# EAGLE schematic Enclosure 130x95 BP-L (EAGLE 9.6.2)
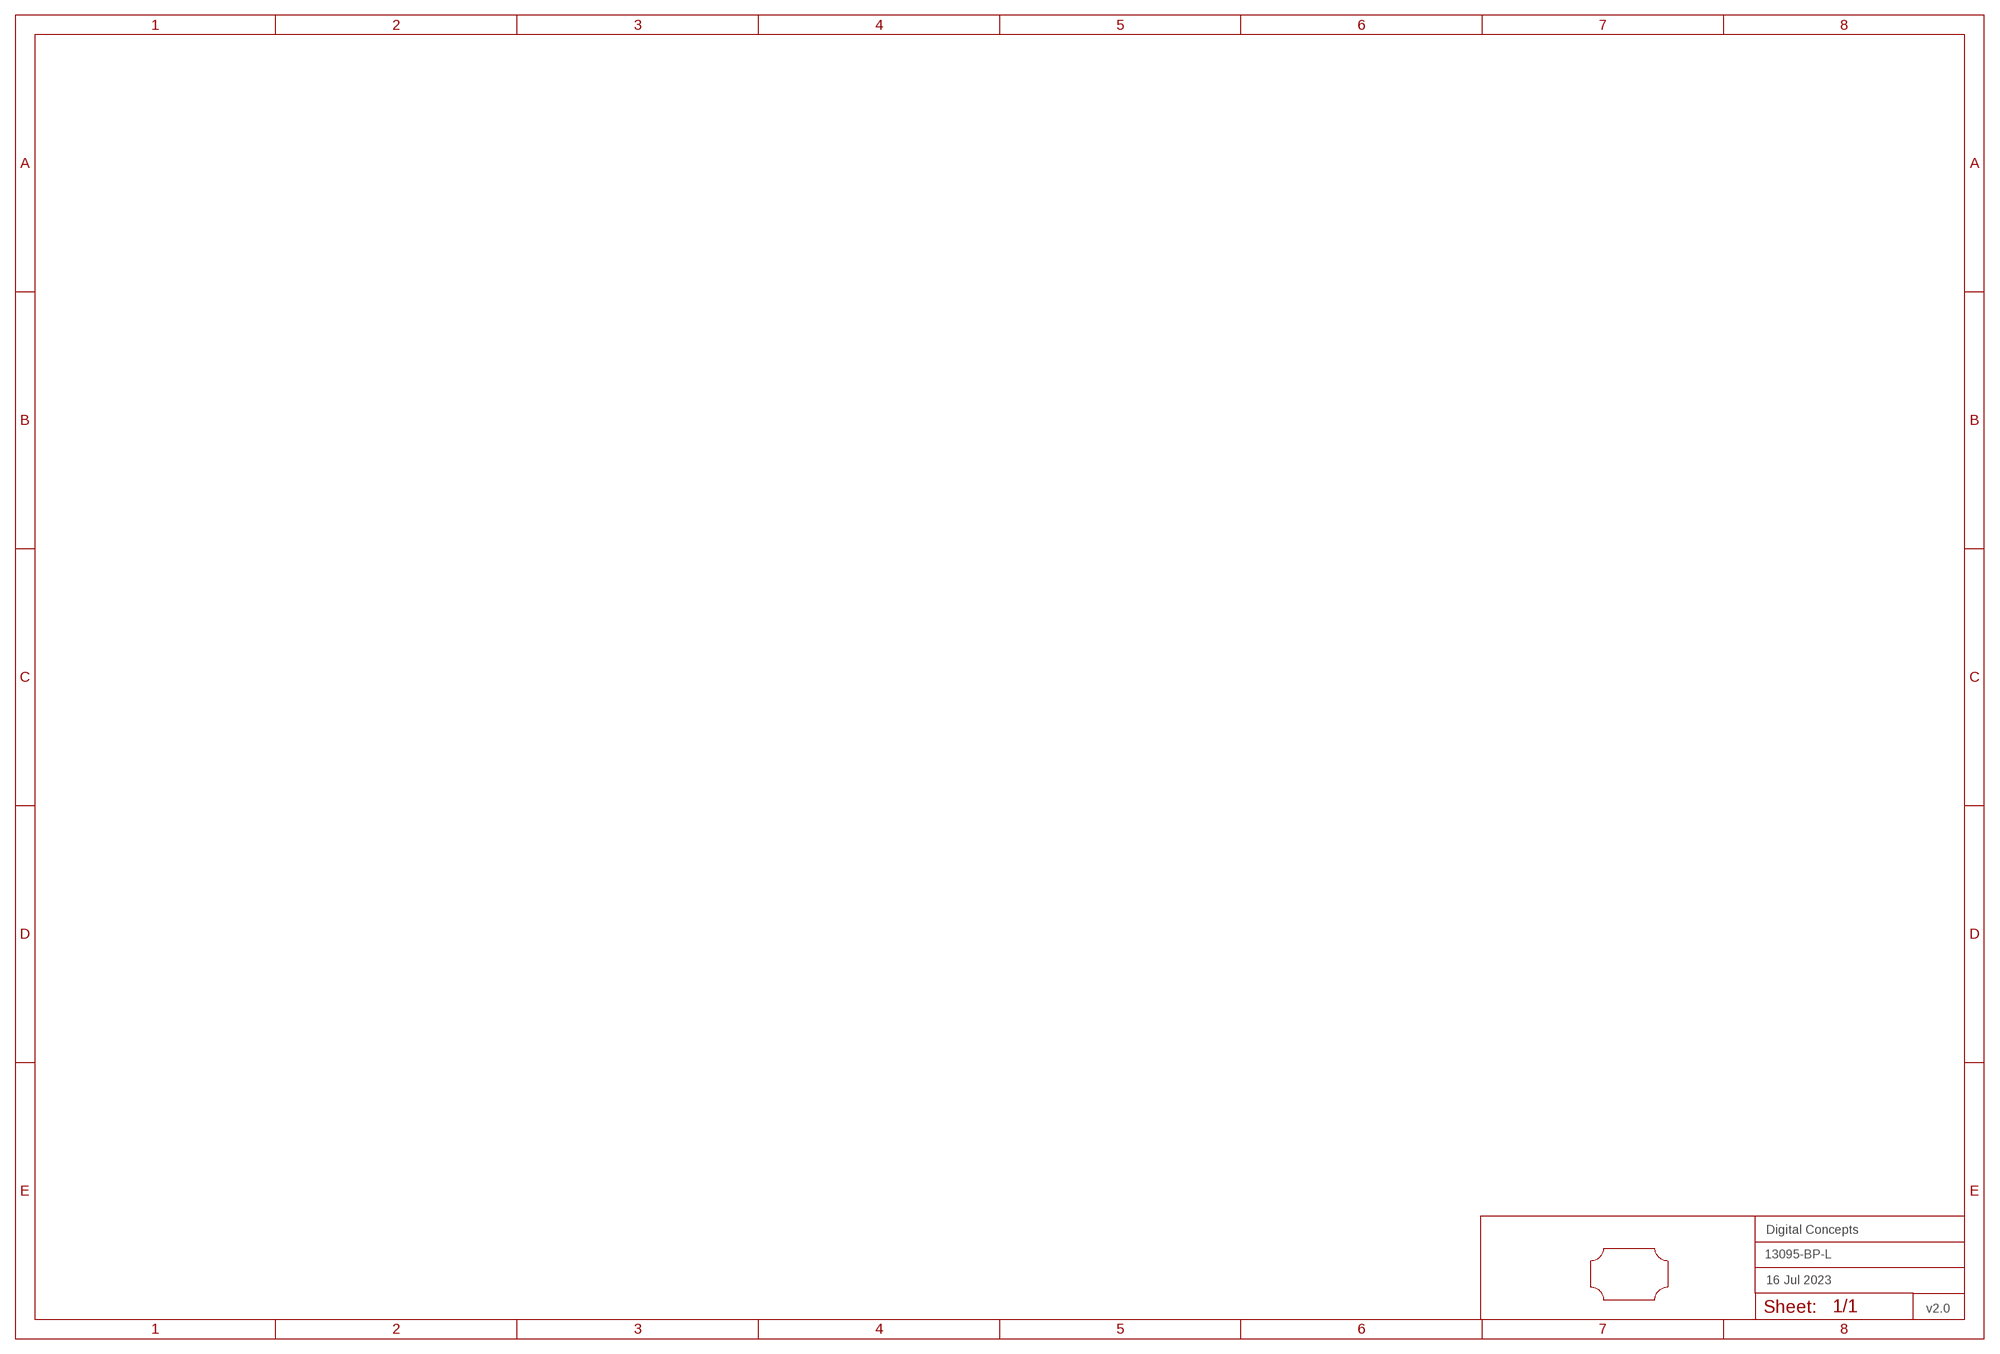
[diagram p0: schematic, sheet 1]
FRAME2 (A3L-LOC): DATE: 16 Jul 2023; OWNER: Digital Concepts; TITLE: 13095-BP-L; VERSION: v2.0

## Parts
U$1  PCB-OUTLINE-130X95-MAX-LC-H2  [PROTO-130X95-OUTLINE-MAX-LC-H2]

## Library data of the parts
U$1 = digitalconcepts:PCB-OUTLINE-130X95-MAX-LC-H2: PCB Eagle Max-Left-Cropped outline for 130 x 95 enclosure (Horizontal format)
